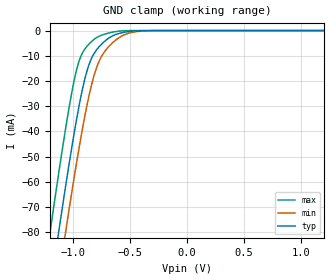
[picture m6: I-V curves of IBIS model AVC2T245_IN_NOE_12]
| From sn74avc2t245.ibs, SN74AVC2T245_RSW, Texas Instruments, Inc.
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[Model]   AVC2T245_IN_NOE_12
Model_type  Input
Vinl=0.385
Vinh=0.845
| variable   typ   min   max
C_comp   2.83pF   2.28pF   3.31pF
[Temperature Range]   40   100   -40
| Ambient temperature   25   85   -40
[Voltage range]   1.2   1.1   1.3
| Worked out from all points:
|   GND clamp passes 1 mA (typ) near -0.58 V on its own axis
[GND Clamp]
| AVC2T245_IN_NOE_12
|   Voltage   I(typ)   I(min)   I(max)
-4.6V     -1.266A    -1.277A    -1.254A
-1.22V    -108.9mA   -127.3mA   -85.71mA
-1.195V   -101.1mA   -119.4mA   -77.82mA
-1.13V    -81mA      -99.35mA   -57.75mA
-1.065V   -61.6mA    -79.78mA   -38.73mA
-960mV    -32.94mA   -49.96mA   -14.03mA
-905mV    -20.72mA   -35.89mA   -7.898mA
-860mV    -13.49mA   -25.81mA   -5.335mA
-760mV    -5.854mA   -11.09mA   -2.009mA
-615mV    -1.4mA     -3.395mA   -339.9uA
-340mV    -6.933uA   -59.17uA   -50.62nA
1.2V      105.6pA    10.37nA    15.63pA
